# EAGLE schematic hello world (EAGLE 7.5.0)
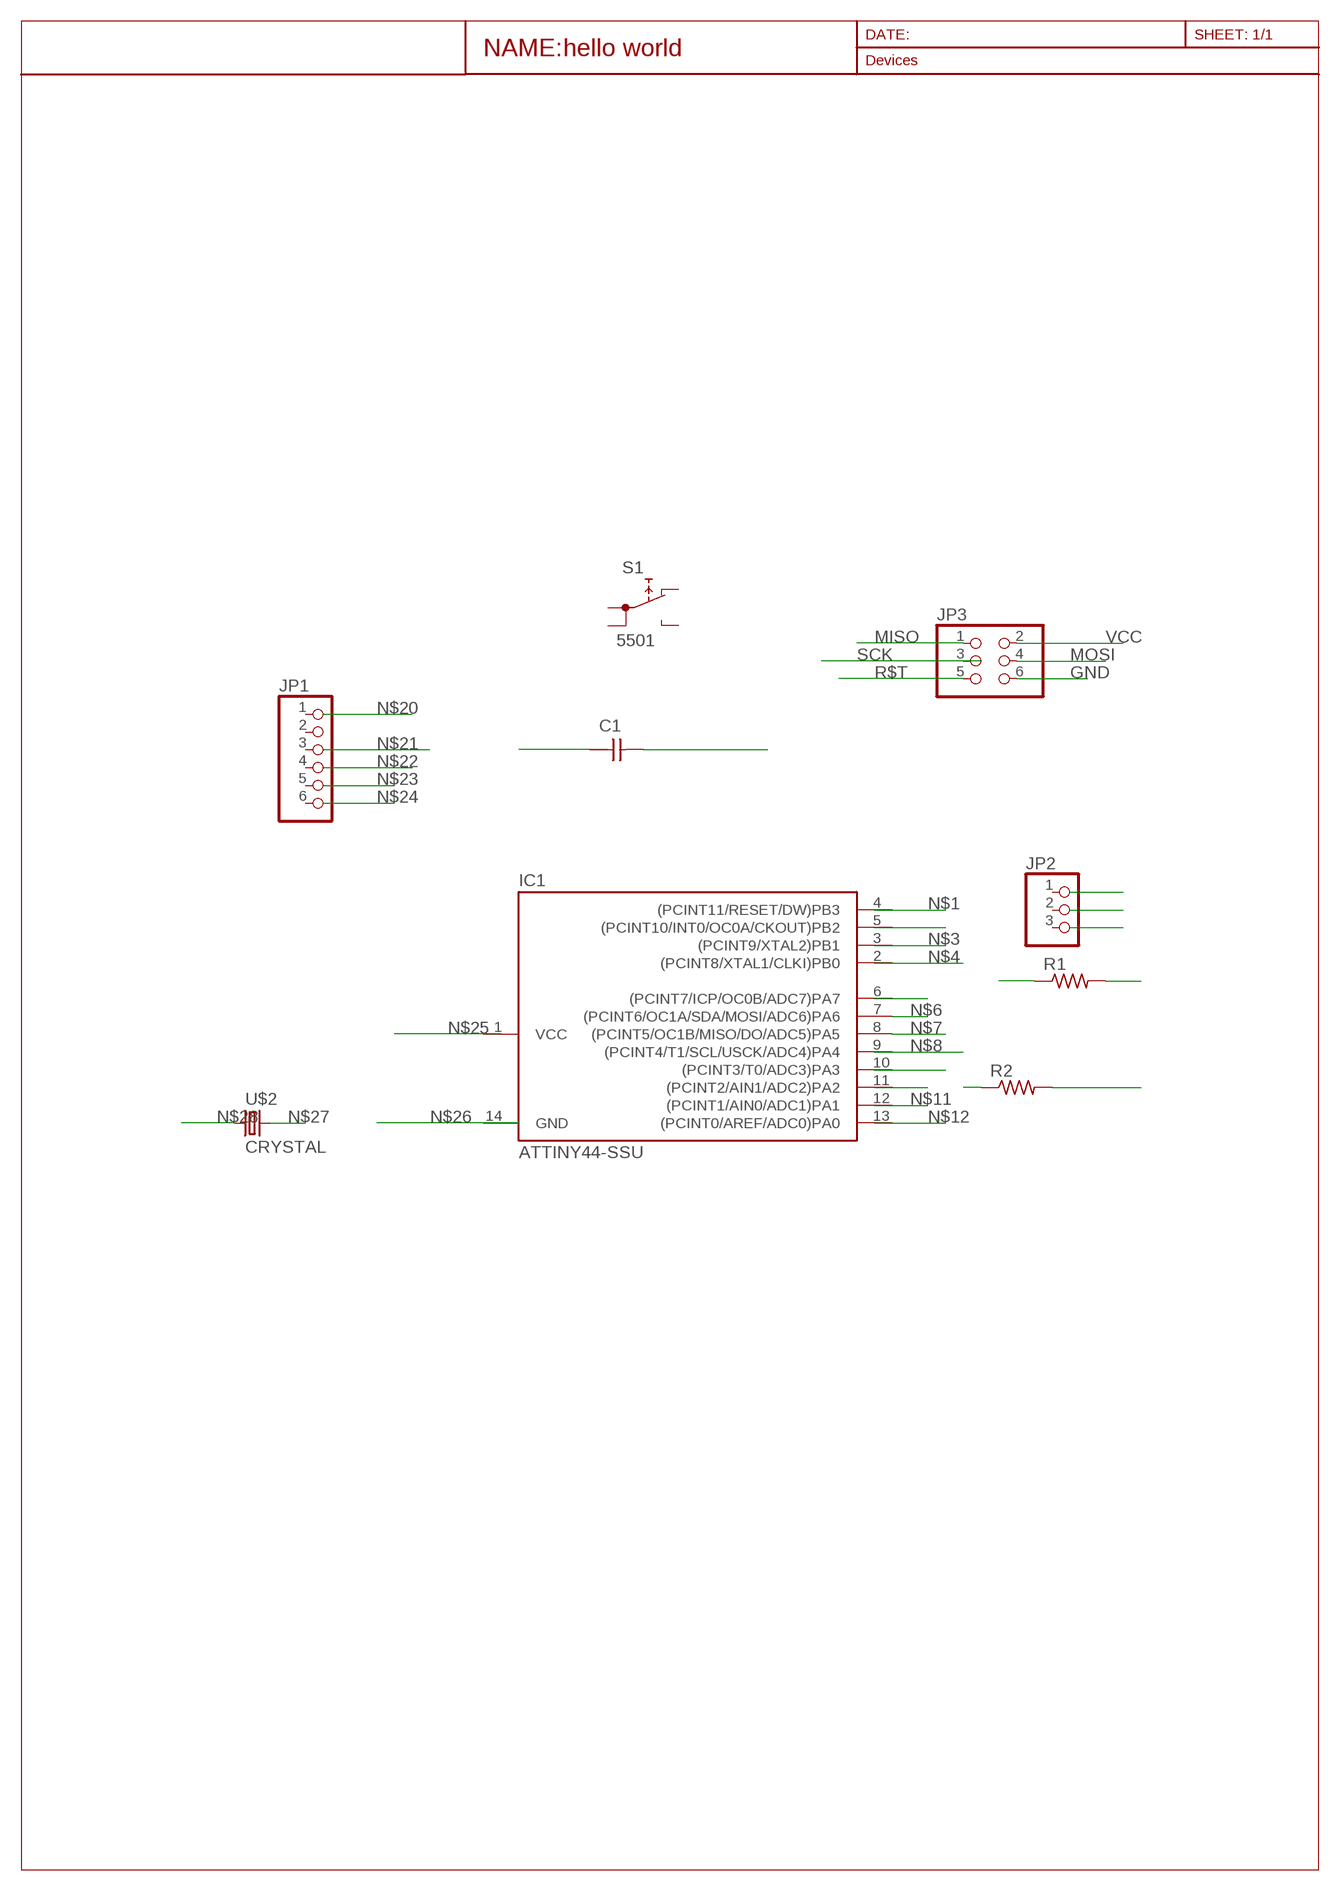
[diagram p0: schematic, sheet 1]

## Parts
C1  CAP-UNPOLARIZEDFAB  [C1206FAB]
IC1  ATTINY44-SSU  [SOIC14]
JP1  PINHD-1X6  [1X06]
JP2  PINHD-1X3  [1X03]
JP3  PINHD-2X3-SMD  [2X03SMD]
R1  RES-US1206FAB  [R1206FAB]
R2  RES-US1206FAB  [R1206FAB]
S1  5501  [5501]
U$2  CRYSTAL  [2-SMD-5X3MM]

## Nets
GND: JP3.6
MISO: JP3.1
MOSI: JP3.4
N$6: IC1.7((PCINT6/OC1A/SDA/MOSI/ADC6)PA6)
N$7: IC1.8((PCINT5/OC1B/MISO/DO/ADC5)PA5)
N$13: R2.2
N$14: R2.1
N$15: R1.2
N$16: R1.1
N$27: U$2.P$2
N$28: U$2.P$1
N$29: C1.2
R$T: JP3.5
VCC: JP3.2
Unconnected: C1.1 IC1.2((PCINT8/XTAL1/CLKI)PB0) IC1.3((PCINT9/XTAL2)PB1) IC1.4((PCINT11/RESET/DW)PB3) IC1.5((PCINT10/INT0/OC0A/CKOUT)PB2) IC1.6((PCINT7/ICP/OC0B/ADC7)PA7) IC1.9((PCINT4/T1/SCL/USCK/ADC4)PA4) IC1.10((PCINT3/T0/ADC3)PA3) IC1.11((PCINT2/AIN1/ADC2)PA2) IC1.12((PCINT1/AIN0/ADC1)PA1) IC1.13((PCINT0/AREF/ADC0)PA0) JP1.1 JP1.2 JP1.3 JP1.4 JP1.5 JP1.6 JP2.1 JP2.2 JP2.3 JP3.3 S1.1A S1.1B S1.NC S1.NO

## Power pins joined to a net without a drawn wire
GND: IC1.14(GND)
VCC: IC1.1(VCC)

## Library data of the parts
C1 = fab (1):CAP-UNPOLARIZED
IC1 = fab (1):ATTINY44
JP1 = pinhead:PINHD-1X6: PIN HEADER
JP2 = pinhead:PINHD-1X3: PIN HEADER
JP3 = fab (1):PINHD-2X3-SMD: PIN HEADER
R1 R2 = fab (1):RES-US: Resistor (US Symbol)
S1 = switch:55?: PUSHBUTTON SERIES 5500 SWITCHES Source: www.e-switch.com .. 5500.pdf
U$2 = fab (1):CRYSTAL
